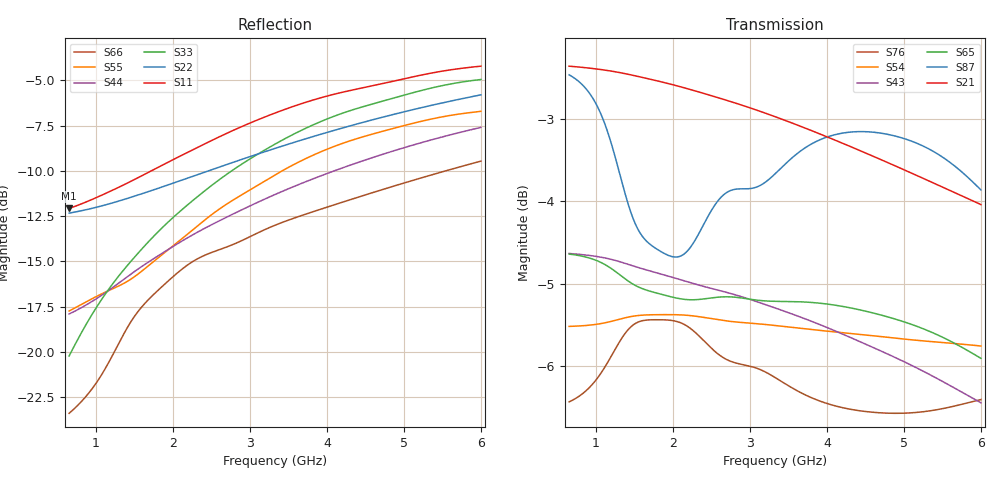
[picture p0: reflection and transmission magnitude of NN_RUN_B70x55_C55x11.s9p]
! IGNION VIRTUAL ANTENNA LIBRARY
! NN_RUN_B70x55_C55x11
! Virtual Antenna™ RUN mXTEND™: NN02-224 12.0 mm x 3.0 mm x 2.4 mm
! https://ignion.io/product/run-mxtend/
! Board: 70 mm x 55 mm
! Clearance Area: 55 mm x 11 mm
! Feeding line: L-shape; 11mm x 2mm and 5mm x 2mm
! Applications: Fleet management, IoT
! Frequency range 0.65GHz to 6GHz, step 10MHz
! Number of ports 9
! This product and its use is protected by at least one or more of the following patents and patent
! applications US 8,203,492 B2; US 8,237,615 B2; PCT/EP2013/064692; WO 2014/012842 A1; US 2019/190122 A1;
! US 62/072,671; and other domestic and international patents pending. Additional information about
! patents related to this product is available at https://ignion.io/files/Patent-list-NN.pdf, all
! rights reserved. Copyright, Ignion 2021.
! Need more help? Your platform is much different than these examples in the manual? Use our
! Fast Track service (https://ignion.io/fast-track/), for free, and get a personalized antenna design in
! just 24 hours.
! Touchstone port 1 = "Series Port"
! Touchstone port 2 = "Shunt Port"
! Touchstone port 3 = "Series Port"
! Touchstone port 4 = "Shunt Port"
! Touchstone port 5 = "Series Port"
! Touchstone port 6 = "Shunt Port"
! Touchstone port 7 = "Series Port"
! Touchstone port 8 = "Shunt Port"
! Touchstone port 9 = "Series Port"
! IE3D S-Parameters Output Version 2.0
# GHZ S MA R 50
! Nport = 9
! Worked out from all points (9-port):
!   536 points, 650 MHz to 6 GHz, reference 50 ohm
!   strongest paths, dB at 650 MHz, 1.99 GHz, 3.33 GHz, 4.67 GHz, 6 GHz:
!     S21: -2.4, -2.6, -3.0, -3.5, -4.0
!     S87: -2.5, -4.7, -3.7, -3.2, -3.9
!     S65: -4.6, -5.2, -5.2, -5.4, -5.9
!     S43: -4.6, -4.9, -5.3, -5.8, -6.4
!     S54: -5.5, -5.4, -5.5, -5.6, -5.8
!     S76: -6.4, -5.4, -6.1, -6.6, -6.4
!   lowest |S11| = -12.1 dB at 650 MHz (marker M1), VSWR 1.66, Z = 31.1 + j7.45 ohm
!   |S11| at or under -10 dB: start of sweep to 1.717 GHz
